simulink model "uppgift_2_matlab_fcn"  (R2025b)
settings: Solver=VariableStepAuto  StartTime=0.0  StopTime=10.0  RelTol=1e-3
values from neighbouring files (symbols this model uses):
  m_th_1 = 12/1000    (= 0.012)    [Lektion_2.m]
  m_th_2 = 16/1000    (= 0.016)    [Lektion_2.m]
  tau_th = 1/0.1    (= 10)    [Lektion_2.m]

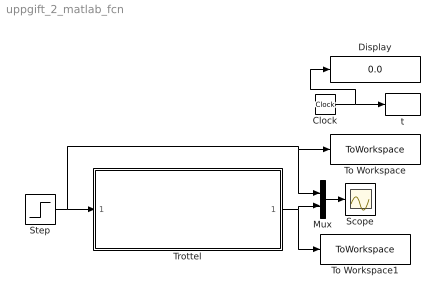
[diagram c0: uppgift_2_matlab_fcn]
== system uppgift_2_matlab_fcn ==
  Clock : Clock
  Display : Display
  Mux : Mux  Inputs=2
  Scope : Scope
  Step : Step  Time=2  Before=m_th_1  After=m_th_2  SampleTime=0
  To Workspace : ToWorkspace  VariableName=m_at_ref  SampleTime=-1
  To Workspace1 : ToWorkspace  VariableName=m_at  SampleTime=-1
  Trottel : Subsystem
  t : ToWorkspace  VariableName=time  SampleTime=-1
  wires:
  Step/1 -> To Workspace/1, Mux/1, Trottel/1(m_at,raf [kg/s])
  Mux/1 -> Scope/1
  Trottel/1(m_at [kg/s]) -> To Workspace1/1, Mux/2
  Clock/1 -> t/1, Display/1

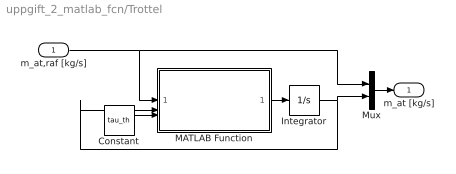
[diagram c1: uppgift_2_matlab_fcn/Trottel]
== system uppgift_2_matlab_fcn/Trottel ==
  m_at,raf [kg/s] : Inport
  Constant : Constant  Value=tau_th
  Integrator : Integrator  InitialCondition=m_th_1
  MATLAB Function : MATLAB Function  TreatAsAtomicUnit=on
  Mux : Mux  Inputs=2
  m_at [kg/s] : Outport
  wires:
  Integrator/1 -> MATLAB Function/2(actual), Mux/2
  Mux/1 -> m_at [kg/s]/1
  m_at,raf [kg/s]/1 -> MATLAB Function/1(ref), Mux/1
  MATLAB Function/1(alpha) -> Integrator/1
  Constant/1 -> MATLAB Function/3(tau)

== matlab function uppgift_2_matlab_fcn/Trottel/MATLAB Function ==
function alpha = fcn(ref, actual, tau)
error = ref - actual;

alpha =  error*tau;
